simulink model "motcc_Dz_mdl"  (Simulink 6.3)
settings: Solver=ode45  StartTime=0.0  StopTime=10.0  RelTol=1e-3
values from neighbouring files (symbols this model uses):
  bm = 0.02*N*m*sec/rad    (= 0.02)    [motcc.m]
  Cr = 0*N*m    (= 0)    [motcc.m]
  Ia_0 = 0*A    (= 0)    [motcc.m]
  Ia_max = 100000*A    (= 100000)    [motcc.m]
  Jm = 0.5*Kg*m^2    (= 0.5)    [motcc.m]
  K = (1/Ep-1)/dcgain(gs)    [motcc.m]
  Km = 1    [motcc.m]
  La = 10*mHenry    (= 0.01)    [motcc.m]
  Ra = 2*Ohm    (= 2)    [motcc.m]
  Tc = Tfin/2000    (= 5e-05)    [motcc.m]
  Va_max = 10000000*V    (= 10000000)    [motcc.m]
  Wm_0 = 0*rpm    (= 0)    [motcc.m]
  Wref = 600*rpm    (= 62.8318530718)    [motcc.m]
undefined symbols (not defined in the file or in its folder): den, num, Tsamp

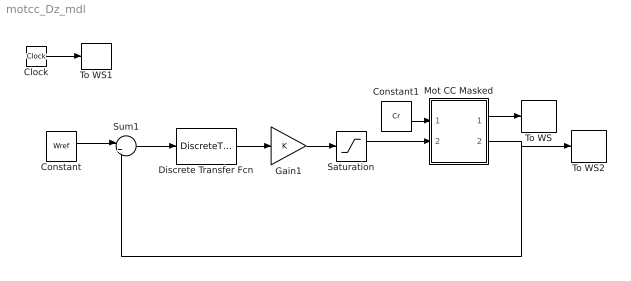
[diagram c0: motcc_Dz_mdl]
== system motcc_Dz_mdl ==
  Clock : Clock
  Constant : Constant  Value=Wref
  Constant1 : Constant  Value=Cr
  Discrete Transfer Fcn : DiscreteTransferFcn  Numerator=num  Denominator=den  SampleTime=Tsamp
  Gain1 : Gain  Gain=K
  Mot CC Masked : Subsystem  mask(Motore in corrente continua){La=La, Ra=Ra, Km=Km, Jm=Jm, bm=bm, Ia_max=Ia_max}
      mask prompts: La "Induttanza di armature La [H]"; Ra "Resistenza di armatura Ra [0hm]"; Km "Costante di coppia Km"; Jm "Inerzia del motore  Jm"; bm "Coefficiente di attrito bm"; Ia_max "Corrente massima Ia_max"
      mask help: Parametri elettrici: La, Ra, Ia_max Parametri meccanici: Jm, bm
  Saturation : Saturate  UpperLimit=Va_max  LowerLimit=-Va_max
  Sum1 : Sum  Inputs=|+-
  To WS : ToWorkspace  VariableName=Ia  SampleTime=Tc  SaveFormat=Array
  To WS1 : ToWorkspace  VariableName=t  SampleTime=Tc  SaveFormat=Array
  To WS2 : ToWorkspace  VariableName=Wm  SampleTime=Tc  SaveFormat=Array
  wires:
  Clock/1 -> To WS1/1
  Constant1/1 -> Mot CC Masked/1(Tr)
  Mot CC Masked/1(Ia) -> To WS/1
  Mot CC Masked/2(Wm) -> To WS2/1, Sum1/2
  Constant/1 -> Sum1/1
  Sum1/1 -> Discrete Transfer Fcn/1
  Gain1/1 -> Saturation/1
  Saturation/1 -> Mot CC Masked/2(Va)
  Discrete Transfer Fcn/1 -> Gain1/1

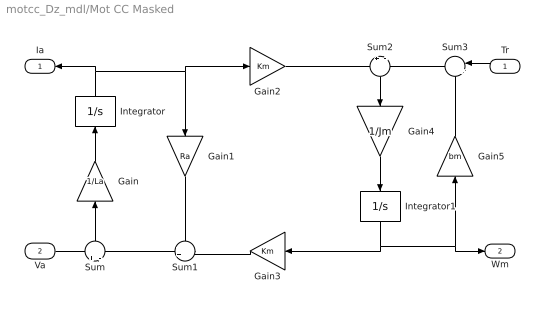
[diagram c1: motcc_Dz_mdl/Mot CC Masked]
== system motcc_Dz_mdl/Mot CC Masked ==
  Tr : Inport  Orientation=left
  Va : Inport  Port=2
  Gain : Gain  Orientation=up  Gain=1/La
  Gain1 : Gain  Orientation=down  Gain=Ra
  Gain2 : Gain  Gain=Km
  Gain3 : Gain  Orientation=left  Gain=Km
  Gain4 : Gain  Orientation=down  Gain=1/Jm
  Gain5 : Gain  Orientation=up  Gain=bm
  Integrator : Integrator  Orientation=up  InitialCondition=Ia_0  LimitOutput=on  UpperSaturationLimit=Ia_max  LowerSaturationLimit=-Ia_max
  Integrator1 : Integrator  Orientation=down  InitialCondition=Wm_0
  Sum : Sum  Orientation=up  Inputs=+|-
  Sum1 : Sum  Inputs=++|
  Sum2 : Sum  Orientation=down  Inputs=+|-
  Sum3 : Sum  Orientation=left  Inputs=|++
  Ia : Outport  Orientation=left
  Wm : Outport  Port=2
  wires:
  Sum/1 -> Gain/1
  Gain/1 -> Integrator/1
  Integrator/1 -> Gain1/1, Gain2/1, Ia/1
  Sum1/1 -> Sum/2
  Gain1/1 -> Sum1/1
  Gain3/1 -> Sum1/2
  Gain2/1 -> Sum2/1
  Sum2/1 -> Gain4/1
  Gain4/1 -> Integrator1/1
  Integrator1/1 -> Gain3/1, Gain5/1, Wm/1
  Gain5/1 -> Sum3/2
  Sum3/1 -> Sum2/2
  Tr/1 -> Sum3/1
  Va/1 -> Sum/1
